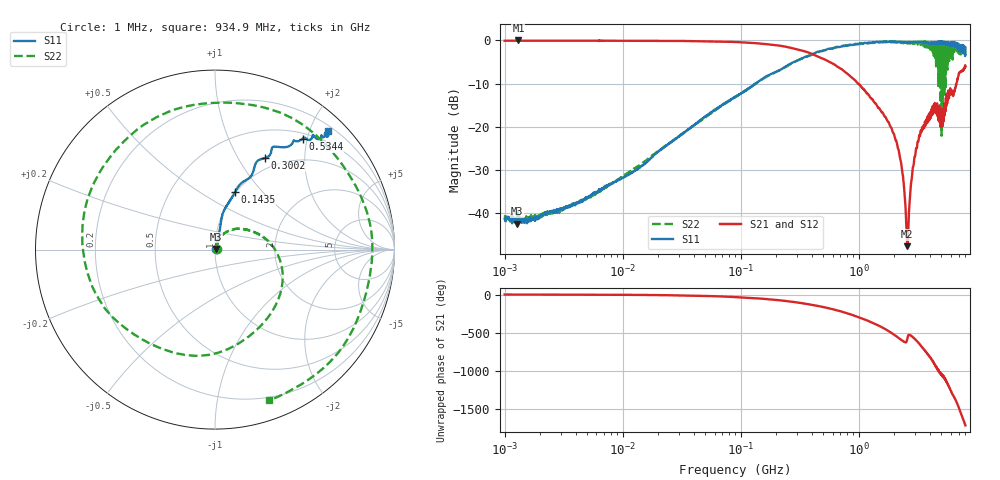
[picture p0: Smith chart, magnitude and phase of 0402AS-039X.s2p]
!s-Parameter Generated by FASTRON Sdn. Bhd.
!FASTRON P/N : 0402AS-039X
!Keysight Technologies: E5071C_MY46733604_B.14.02
!Date: Mon Dec 01 10:46:18 2025
!Version  :Rev00  Mon Dec 01 10:46:18 2025
!Data & Calibration Information:
!Freq  S11:SOLT2(ON)  S21:SOLT2(ON)  S12:SOLT2(ON)  S22:SOLT2(ON)
!PortZ  Port1:50+j0  Port2:50+j0
!When reading reference impedance value at option line is always used.
! Remarks : This data is being provided solely for informational purposes.
# Hz S dB R 50
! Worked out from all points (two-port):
!   1601 points, 1 MHz to 8 GHz, reference 50 ohm
!   highest |S21| = -0.02 dB at 1.31 MHz (marker M1); lowest = -47.7 dB at 2.575 GHz (marker M2)
!   |S21| within 3 dB of the highest: start of sweep to 391.3 MHz
!   lowest |S11| = -42.5 dB at 1.277 MHz (marker M3), VSWR 1.02, Z = 50.7 + j0.284 ohm
!   |S11| at or under -10 dB: start of sweep to 133.7 MHz
!   |S22| runs from -42.2 to -0.2 dB; largest |S21 - S12| = 0.027
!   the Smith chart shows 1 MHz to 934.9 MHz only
!   S11 on the Smith chart (normalised r, x): 1 MHz: 1.02, +0.01; 143.5 MHz: 0.99, +0.72; 300.2 MHz: 0.85, +1.31; 534.4 MHz: 0.59, +1.92; 934.9 MHz: 0.30, +2.31
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1000000  -41.40 21.0  -0.08 -0.4  -0.07 -0.4  -40.80 21.9
1277234  -42.50 21.9  -0.09 -0.6  -0.07 -0.6  -41.70 15.1
1310238  -40.50 24.3  -0.02 -0.6  -0.08 -0.5  -40.80 12.8
4479405  -37.00 56.3  -0.08 -1.8  -0.07 -1.8  -37.20 56.9
2.00676e7  -25.70 74.3  -0.10 -7.6  -0.10 -7.5  -25.70 69.3
8.994653e7  -13.10 77.2  -0.38 -32.9  -0.37 -32.9  -13.10 28.9
1.435152e8  -9.41 70.8  -0.72 -51.8  -0.72 -51.7  -9.47 -0.5
3.00191e8  -4.72 61.4  -2.09 -104.0  -2.08 -104.0  -4.67 -92.0
4.006501e8  -3.33 56.8  -3.13 -135.0  -3.12 -135.0  -3.24 -149.0
5.344419e8  -2.08 51.7  -4.65 -173.0  -4.63 -174.0  -2.17 139.0
9.348876e8  -0.80 46.3  -9.33 79.2  -9.33 79.1  -0.98 -70.2
1.341815e9  -0.43 53.1  -14.20 -17.2  -14.20 -17.3  -0.53 88.4
1.542898e9  -0.34 58.9  -16.40 -62.0  -16.40 -62.2  -0.38 -7.5
1.7949e9  -0.27 65.4  -19.00 -119.0  -19.00 -119.0  -0.42 -129.0
2.061212e9  -0.42 71.3  -23.20 -180.0  -23.20 -180.0  -0.36 102.0
2.252141e9  -0.51 74.3  -27.60 137.0  -27.60 137.0  -0.38 8.1
2.57493e9  -0.42 82.5  -47.70 136.0  -47.50 137.0  -0.73 -153.0
3.000426e9  -0.43 93.7  -26.80 135.0  -26.80 135.0  -0.41 2.8
3.365624e9  -0.38 103.0  -21.10 46.3  -21.00 46.0  -1.02 172.0
3.730463e9  -0.67 111.0  -18.30 -33.8  -18.30 -34.3  -1.17 8.4
4.115571e9  -0.78 121.0  -16.00 -120.0  -16.00 -120.0  -1.24 -169.0
8e9  -1.67 -111.0  -6.01 89.7  -6.02 89.3  -3.60 126.0
